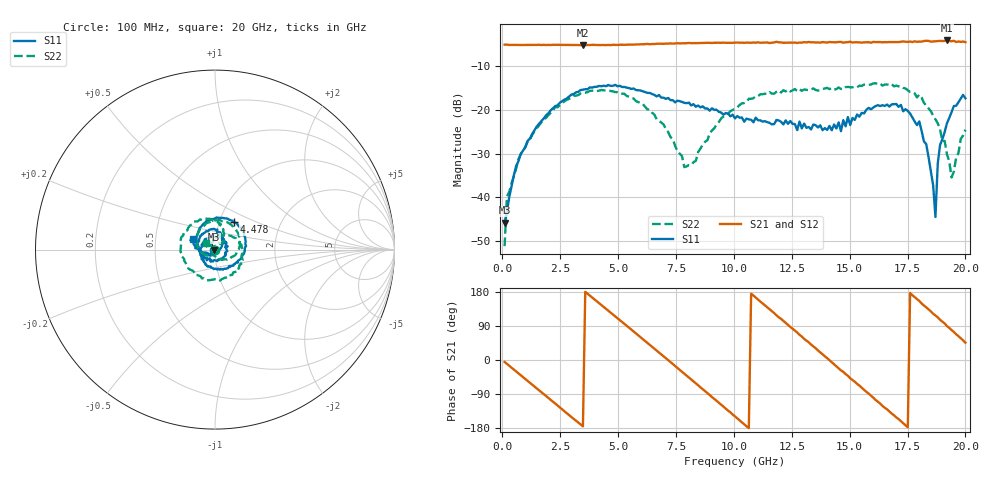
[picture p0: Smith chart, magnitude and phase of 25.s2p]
!Agilent Technologies,N5230C,MY49001569,A.09.33.09
!Agilent N5230C: A.09.33.09
!Date: Tuesday, July 28, 2015 14:53:52
!Correction: S11(Full 2 Port(1,2))
!S21(Full 2 Port(1,2))
!S12(Full 2 Port(1,2))
!S22(Full 2 Port(1,2))
!S2P File: Measurements: S11, S21, S12, S22:
# Hz S  dB  R 50
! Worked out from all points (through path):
!   201 points, 100 MHz to 20 GHz, reference 50 ohm
!   highest |S21| = -4.24 dB at 19.2 GHz (marker M1); lowest = -5.3 dB at 3.483 GHz (marker M2)
!   group delay of S21, straight-line fit = 143 ps
!   lowest |S11| = -45.8 dB at 100 MHz (marker M3), VSWR 1.01, Z = 49.5 - j0.125 ohm
!   |S11| at or under -10 dB: start of sweep to end of sweep
!   |S22| runs from -51.1 to -14.0 dB; largest |S21 - S12| = 0.024
!   S11 on the Smith chart (normalised r, x): 100 MHz: 0.99, -0.00; 4.478 GHz: 1.17, +0.37; 20 GHz: 0.78, +0.09
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1e8  -45.76 -165.9  -5.20 -5.2  -5.18 -5.6  -51.11 -14.5
1.995e8  -43.36 -47.2  -5.19 -10.1  -5.22 -10.4  -39.81 -27.8
7.965e8  -30.08 -110.5  -5.28 -40.1  -5.26 -40.3  -30.10 -109.8
1.9905e9  -20.83 176.4  -5.25 -100.3  -5.28 -100.3  -21.27 179.2
3.483e9  -15.46 100.4  -5.32 -175.1  -5.30 -175.1  -16.14 104.4
4.478e9  -14.67 55.4  -5.29 135.1  -5.32 134.9  -15.67 57.0
5.5725e9  -15.29 11.0  -5.19 80.3  -5.18 80.0  -17.33 5.1
6.7665e9  -16.68 -29.1  -4.98 20.0  -5.00 19.6  -22.64 -47.7
7.861e9  -18.46 -62.7  -4.90 -36.1  -4.90 -36.2  -33.11 -132.0
8.9555e9  -20.24 -104.3  -4.78 -92.2  -4.77 -92.9  -25.43 100.4
1.005e10  -22.00 -167.5  -4.73 -148.7  -4.75 -149.3  -19.82 52.7
1.1841e10  -22.35 72.8  -4.54 117.9  -4.80 117.9  -15.92 -18.0
1.3433e10  -23.39 -29.2  -4.66 35.8  -4.77 34.9  -15.16 -80.7
1.45275e10  -22.92 -109.1  -4.58 -21.6  -4.61 -21.2  -14.94 -129.1
1.5423e10  -21.61 -179.6  -4.68 -67.6  -4.57 -69.1  -14.54 -168.2
1.67165e10  -19.31 110.2  -4.61 -135.8  -4.64 -136.5  -14.37 131.7
1.801e10  -22.69 29.8  -4.50 155.9  -4.50 153.8  -16.58 78.9
1.87065e10  -44.47 -66.8  -4.45 117.4  -4.42 116.8  -22.22 54.8
1.8806e10  -32.32 -130.3  -4.39 112.6  -4.35 110.3  -23.11 44.0
1.9204e10  -23.11 -165.9  -4.24 89.5  -4.46 89.6  -30.21 65.3
1.9403e10  -20.58 177.4  -4.43 79.1  -4.42 77.7  -35.47 88.4
2e10  -17.43 153.7  -4.64 45.7  -4.69 44.9  -24.58 143.5
